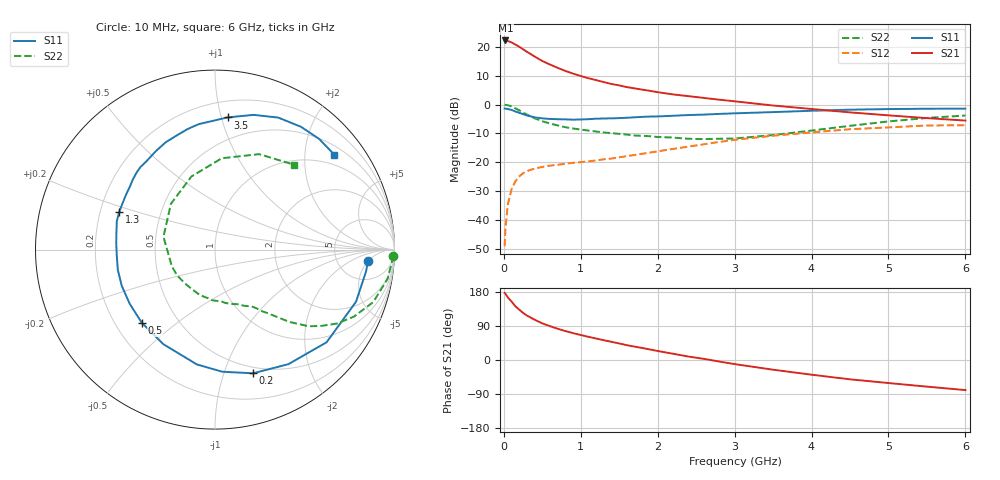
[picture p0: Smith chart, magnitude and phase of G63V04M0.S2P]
! SIEMENS Small Signal Semiconductors
! BFG193
! Si NPN RF Bipolar Junction Transistor in SOT223
! VCE = 3 V  IC = 4 mA
! Common Emitter S-Parameters:  August  1996
# GHz  S  MA  R  50
!  f  S11  S21  S12  S22
! GHz  MAG  ANG  MAG  ANG  MAG  ANG  MAG  ANG
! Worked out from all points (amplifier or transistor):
!   36 points, 10 MHz to 6 GHz, reference 50 ohm
!   highest |S21| = 22.2 dB at 20 MHz (marker M1)
!   |S21| within 3 dB of that: start of sweep to 246.7 MHz
!   unconditionally stable (mu >= 1): 1.204 GHz to 2.608 GHz
!   at 250 MHz: K = 0.29, MSG = 21.5 dB, |S12| = -23.8 dB
!   at 1.4 GHz: K = 1.08, MAG = 11.2 dB, |S12| = -18.7 dB
!   at 6 GHz: K = 0.90, MSG = 0.8 dB, |S12| = -7.2 dB
!   S11 on the Smith chart (normalised r, x): 10 MHz: 11, -5; 200 MHz: 0.44, -1.26; 500 MHz: 0.31, -0.38; 1.3 GHz: 0.28, +0.18; 3.5 GHz: 0.32, +1.05; 6 GHz: 0.71, +2.70
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0.01  0.8548 -4.1  12.84 177.0  0.0035 93.0  0.9922 -2.0
0.02  0.8505 -8.2  12.94 175.1  0.0067 84.4  0.9881 -3.9
0.05  0.8377 -20.3  12.68 165.6  0.018 78.7  0.9753 -9.6
0.1  0.8082 -39.7  11.97 154.3  0.0339 70.5  0.9292 -18.3
0.15  0.7582 -57.3  11 141.8  0.0468 60.9  0.8599 -25.7
0.2  0.7211 -72.9  10.06 132.9  0.0567 55.2  0.7949 -31.2
0.25  0.6816 -86.6  9.1 124.3  0.0644 49.3  0.726 -35.9
0.3  0.6476 -99.0  8.237 117.3  0.0701 45.5  0.6724 -39.4
0.4  0.6005 -118.6  6.812 106.4  0.0777 39.8  0.578 -44.2
0.5  0.5766 -135.0  5.696 96.7  0.0829 36.0  0.5137 -47.2
0.6  0.563 -147.6  4.946 89.2  0.0871 34.6  0.4695 -49.7
0.7  0.5574 -158.8  4.338 82.4  0.0903 33.4  0.4347 -52.4
0.9  0.5483 -176.1  3.443 70.9  0.0976 33.1  0.3842 -56.3
1.1  0.5581 169.7  2.862 61.2  0.1036 33.3  0.3542 -62.2
1.3  0.5735 158.5  2.452 52.2  0.1123 34.3  0.3282 -67.8
1.6  0.5899 143.5  2.008 39.0  0.1276 34.9  0.3017 -79.3
2.2  0.6394 121.2  1.5 16.5  0.1703 32.2  0.2676 -107.8
2.8  0.6888 102.8  1.216 -4.1  0.2249 24.5  0.2553 -145.2
3.5  0.74 84.5  0.963 -25.6  0.2884 9.9  0.296 166.0
4.5  0.8155 64.4  0.732 -51.0  0.3737 -11.2  0.4279 107.9
5.5  0.8467 46.8  0.582 -70.3  0.4333 -37.6  0.5859 65.2
6  0.8495 38.5  0.528 -79.4  0.4389 -52.4  0.6457 47.1
